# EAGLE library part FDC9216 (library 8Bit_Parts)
Dual In Line / Socket
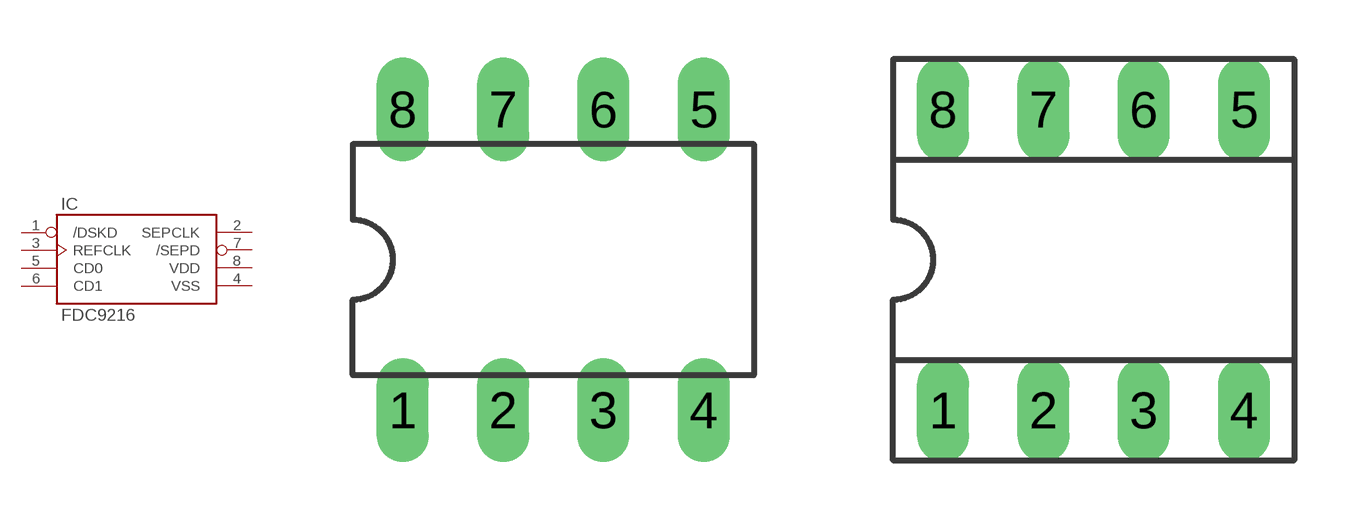
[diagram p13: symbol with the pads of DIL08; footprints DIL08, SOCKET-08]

Designator prefix IC

## FDC9216  [DIL08]
1  /DSKD  in
2  SEPCLK  out
3  REFCLK  pas
4  VSS  pwr
5  CD0  in
6  CD1  in
7  /SEPD  out
8  VDD  pwr

## FDC9216S  [SOCKET-08]
Pads as for DIL08

## Footprint DIL08 (pad centres in mm)
Dual In Line Package
drill 0.813 long: 1 -3.81,-3.81; 2 -1.27,-3.81; 3 1.27,-3.81; 4 3.81,-3.81; 5 3.81,3.81; 6 1.27,3.81; 7 -1.27,3.81; 8 -3.81,3.81

## Footprint SOCKET-08 (pad centres in mm)
Dual In Line Socket
drill 0.813 long: 1 -3.81,-3.81; 2 -1.27,-3.81; 3 1.27,-3.81; 4 3.81,-3.81; 5 3.81,3.81; 6 1.27,3.81; 7 -1.27,3.81; 8 -3.81,3.81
